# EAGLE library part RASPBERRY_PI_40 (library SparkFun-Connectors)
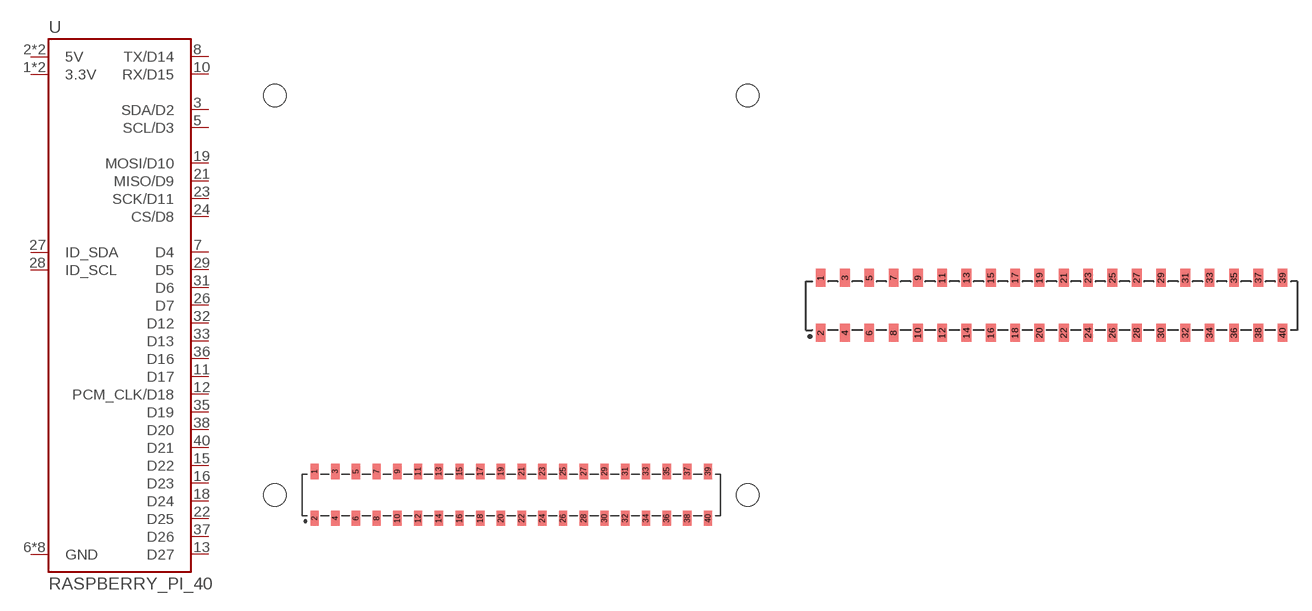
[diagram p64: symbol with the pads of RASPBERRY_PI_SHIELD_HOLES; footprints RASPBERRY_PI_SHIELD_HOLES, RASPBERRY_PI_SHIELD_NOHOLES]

Designator prefix U

## RASPBERRY_PI_40SMD  [RASPBERRY_PI_SHIELD_HOLES]
1  3.3V
2  5V
3  SDA/D2
4  5V
5  SCL/D3
6  GND
7  D4
8  TX/D14
9  GND
10  RX/D15
11  D17
12  PCM_CLK/D18
13  D27
14  GND
15  D22
16  D23
17  3.3V
18  D24
19  MOSI/D10
20  GND
21  MISO/D9
22  D25
23  SCK/D11
24  CS/D8
25  GND
26  D7
27  ID_SDA
28  ID_SCL
29  D5
30  GND
31  D6
32  D12
33  D13
34  GND
35  D19
36  D16
37  D26
38  D20
39  GND
40  D21

## RASPBERRY_PI_40NOHOLES  [RASPBERRY_PI_SHIELD_NOHOLES]
Pads as for RASPBERRY_PI_SHIELD_HOLES

## RASPBERRY_PI_40BTM-NOHOLES (PROD_ID: CONN-13790)  [RASPBERRY_PI_SHIELD_BOTTOM_ENTRY_NOHOLES]
Pads as for RASPBERRY_PI_SHIELD_HOLES

## Footprint RASPBERRY_PI_SHIELD_HOLES (pad centres in mm)
Surface Mount - 2x20 Header Reversed pinout to match Raspberry Pi male header pinout when coupled.
smd 1.02 x 1.87: 1 8.382,7.686; 2 8.382,1.929; 3 10.922,7.686; 4 10.922,1.929; 5 13.462,7.686; 6 13.462,1.929; 7 16.002,7.686; 8 16.002,1.929; 9 18.542,7.686; 10 18.542,1.929; 11 21.082,7.686; 12 21.082,1.929; 13 23.622,7.686; 14 23.622,1.929; 15 26.162,7.686; 16 26.162,1.929; 17 28.702,7.686; 18 28.702,1.929; 19 31.242,7.686; 20 31.242,1.929; 21 33.782,7.686; 22 33.782,1.929; 23 36.322,7.686; 24 36.322,1.929; 25 38.862,7.686; 26 38.862,1.929; 27 41.402,7.686; 28 41.402,1.929; 29 43.942,7.686; 30 43.942,1.929; 31 46.482,7.686; 32 46.482,1.929; 33 49.022,7.686; 34 49.022,1.929; 35 51.562,7.686; 36 51.562,1.929; 37 54.102,7.686; 38 54.102,1.929; 39 56.642,7.686; 40 56.642,1.929
hole 2.75 at 3.512,4.775
hole 2.75 at 61.512,4.775
hole 2.75 at 61.512,53.775
hole 2.75 at 3.512,53.775

## Footprint RASPBERRY_PI_SHIELD_NOHOLES (pad centres in mm)
smd 1.02 x 1.87: 1 8.382,7.686; 2 8.382,1.929; 3 10.922,7.686; 4 10.922,1.929; 5 13.462,7.686; 6 13.462,1.929; 7 16.002,7.686; 8 16.002,1.929; 9 18.542,7.686; 10 18.542,1.929; 11 21.082,7.686; 12 21.082,1.929; 13 23.622,7.686; 14 23.622,1.929; 15 26.162,7.686; 16 26.162,1.929; 17 28.702,7.686; 18 28.702,1.929; 19 31.242,7.686; 20 31.242,1.929; 21 33.782,7.686; 22 33.782,1.929; 23 36.322,7.686; 24 36.322,1.929; 25 38.862,7.686; 26 38.862,1.929; 27 41.402,7.686; 28 41.402,1.929; 29 43.942,7.686; 30 43.942,1.929; 31 46.482,7.686; 32 46.482,1.929; 33 49.022,7.686; 34 49.022,1.929; 35 51.562,7.686; 36 51.562,1.929; 37 54.102,7.686; 38 54.102,1.929; 39 56.642,7.686; 40 56.642,1.929

## Footprint RASPBERRY_PI_SHIELD_BOTTOM_ENTRY_NOHOLES (pad centres in mm)
smd 1.02 x 1.87: 1 8.37,7.665; 2 8.37,1.935; 3 10.91,7.665; 4 10.91,1.935; 5 13.45,7.665; 6 13.45,1.935; 7 15.99,7.665; 8 15.99,1.935; 9 18.53,7.665; 10 18.53,1.935; 11 21.07,7.665; 12 21.07,1.935; 13 23.61,7.665; 14 23.61,1.935; 15 26.15,7.665; 16 26.15,1.935; 17 28.69,7.665; 18 28.69,1.935; 19 31.23,7.665; 20 31.23,1.935; 21 33.77,7.665; 22 33.77,1.935; 23 36.31,7.665; 24 36.31,1.935; 25 38.85,7.665; 26 38.85,1.935; 27 41.39,7.665; 28 41.39,1.935; 29 43.93,7.665; 30 43.93,1.935; 31 46.47,7.665; 32 46.47,1.935; 33 49.01,7.665; 34 49.01,1.935; 35 51.55,7.665; 36 51.55,1.935; 37 54.09,7.665; 38 54.09,1.935; 39 56.63,7.665; 40 56.63,1.935
hole 1.02 at 31.23,6.07
hole 1.02 at 31.23,3.53
hole 1.02 at 28.69,3.53
hole 1.02 at 28.69,6.07
hole 1.02 at 26.15,6.07
hole 1.02 at 26.15,3.53
hole 1.02 at 23.61,3.53
hole 1.02 at 23.61,6.07
hole 1.02 at 36.31,6.07
hole 1.02 at 36.31,3.53
hole 1.02 at 33.77,3.53
hole 1.02 at 33.77,6.07
hole 1.02 at 15.99,6.07
hole 1.02 at 15.99,3.53
hole 1.02 at 13.45,3.53
hole 1.02 at 13.45,6.07
hole 1.02 at 10.91,6.07
hole 1.02 at 10.91,3.53
hole 1.02 at 8.37,3.53
hole 1.02 at 8.37,6.07
hole 1.02 at 21.07,6.07
hole 1.02 at 21.07,3.53
hole 1.02 at 18.53,3.53
hole 1.02 at 18.53,6.07
hole 1.02 at 46.47,6.07
hole 1.02 at 46.47,3.53
hole 1.02 at 43.93,3.53
hole 1.02 at 43.93,6.07
hole 1.02 at 41.39,6.07
hole 1.02 at 41.39,3.53
hole 1.02 at 38.85,3.53
hole 1.02 at 38.85,6.07
hole 1.02 at 51.55,6.07
hole 1.02 at 51.55,3.53
hole 1.02 at 49.01,3.53
hole 1.02 at 49.01,6.07
hole 1.02 at 54.09,6.07
hole 1.02 at 56.63,6.07
hole 1.02 at 56.63,3.53
hole 1.02 at 54.09,3.53
hole 1.8 at 55.36,4.8
hole 1.8 at 9.64,4.8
